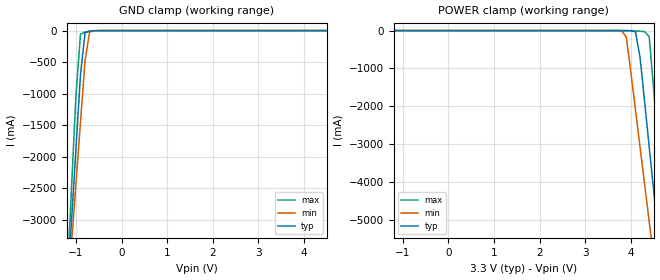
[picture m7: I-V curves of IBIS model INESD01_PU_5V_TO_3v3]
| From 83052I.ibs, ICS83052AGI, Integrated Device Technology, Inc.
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[Model] INESD01_PU_5V_TO_3v3
Model_type   Input
Polarity   Non-Inverting
Vinl = 1.4V
Vinh = 1.85V
|   typ   min   max
C_comp   2pF   1.5pF   2.5pF
|   typ   min   max
[Voltage range]  3.3V   3.135V   3.465V
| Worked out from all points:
|   GND clamp passes 1 mA (typ) near -0.53 V on its own axis
[GND_clamp]
|Voltage   I(typ)   I(min)   I(max)
-3.3V     -29.05A    -25.05A    -35.74A
-1.2V     -4.246A    -4.402A    -4.061A
-1.1V     -3.066A    -3.421A    -2.553A
-1V       -1.886A    -2.44A     -1.044A
-900mV    -707.2mA   -1.46A     -57.45mA
-800mV    -35.64mA   -480.8mA   -24.42mA
-700mV    -7.042mA   -24.07mA   -13.3mA
-600mV    -2.123mA   -1.734mA   -4.923mA
6.6V      64.3uA     84.42uA    57.85uA
[POWER_clamp]
|Voltage   I(typ)   I(min)   I(max)
-3.3V     64.3uA     80.4uA     60.89uA
3.8V      -415.9uA   -8.87mA    -79.9uA
3.9V      -2.123mA   -177.6mA   -256.3uA
4.1V      -35.64mA   -2.097A    -7.435mA
4.2V      -707.2mA   -3.077A    -16.94mA
4.3V      -1.886A    -4.058A    -29.28mA
4.4V      -3.066A    -5.04A     -160.2mA
4.5V      -4.246A    -6.022A    -1.572A
4.6V      -5.426A    -7.005A    -3.08A
4.7V      -6.607A    -7.988A    -4.589A
4.8V      -7.788A    -8.971A    -6.098A
6.6V      -29.05A    -26.68A    -33.25A
